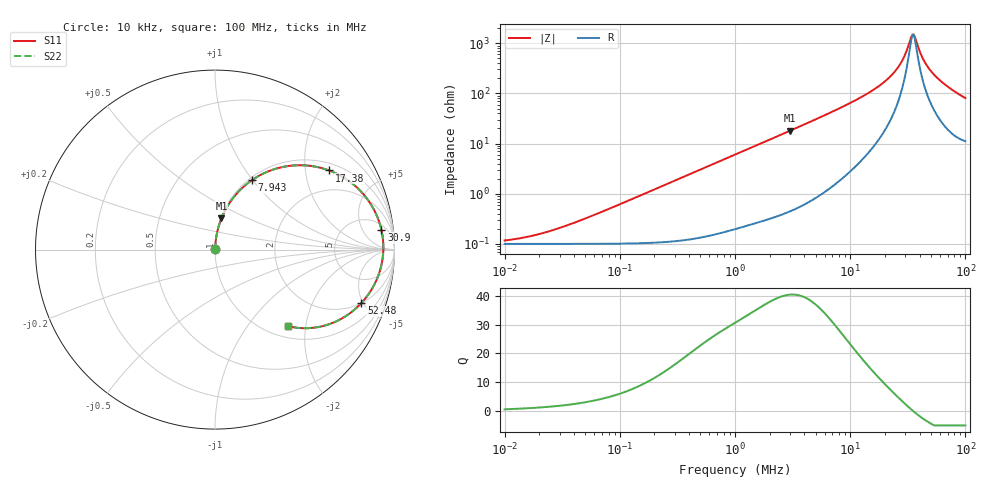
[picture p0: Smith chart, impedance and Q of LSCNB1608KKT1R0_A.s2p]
! LSCNB1608KKT1R0_A  S-PARAMETER MODEL  ( Standard Model )
! Model Generated by TAIYO YUDEN Corporation (http://www.ty-top.com)
! Version 1.0
! TAIYO YUDEN Control No. 170927
! Copyright(c) 2017 TAIYO YUDEN CO.,LTD. All Rights Reserved.
! Product Description (link to TY-COMPAS)
! https://ds.yuden.co.jp/TYCOMPAS/or/detail?pn=LSCNB1608KKT1R0MA&u=M
! Products Name : Inductors
! Characteristics :
!  Inductance : 1.0 [uH] , SRF(min) : - [Hz] , DC Resistance(max) : 123 [mOhm]
!  Rated Current : Saturation  2.0 [A] (dL = 30 [%]), Temp Rise  1.3 [A] (dT = 40 [degC])
!  Case Size : 1.6 x 0.8 / 0.063 x 0.031 [mm/inch] , Thickness : 1.0 / 0.039 [mm/inch]
!  (Conditions: Temperature = 25 [degC] , DC Bias Current = 0 [A])
! External Node Assignments :
!  1  o---GGG---o  2
! GND o---------o GND
! Frequency Range : 10kHz  -  100MHz  [ 402 STEP ]
# MHz S RI R 50
! Freq[MHz].  S11 Real  S11 Imag  S21 Real  S21 Imag  S12 Real  S12 Imag  S22 Real  S22 Imag
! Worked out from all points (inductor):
!   401 points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, 10 kHz to 100 MHz, reference 50 ohm
!   read as one part in series: L = 968 nH near 50.12 kHz
!   highest Q = 40.4 at 3.02 MHz (marker M1), where L = 954 nH
!   self-resonance near 35.2 MHz
!   S11 on the Smith chart (normalised r, x): 10 kHz: 1.00, +0.00; 7.943 MHz: 1.04, +0.99; 17.38 MHz: 1.23, +2.70; 30.9 MHz: 7, +13; 52.48 MHz: 2.01, -4.85; 100 MHz: 1.22, -1.59
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0.01  0.000999 0.000607  0.999 -0.000607  0.999 -0.000607  0.000999 0.000607
0.020417  0.001 0.00124  0.999 -0.00124  0.999 -0.00124  0.001 0.00124
0.046774  0.00101 0.00284  0.999 -0.00284  0.999 -0.00284  0.00101 0.00284
0.218776  0.00125 0.0133  0.9988 -0.0133  0.9988 -0.0133  0.00125 0.0133
1  0.00556 0.0598  0.9944 -0.0598  0.9944 -0.0598  0.00556 0.0598
3.019952  0.0358 0.1738  0.9642 -0.1738  0.9642 -0.1738  0.0358 0.1738
4.677351  0.0799 0.2582  0.9201 -0.2582  0.9201 -0.2582  0.0799 0.2582
7.943282  0.2058 0.387  0.7942 -0.387  0.7942 -0.387  0.2058 0.387
12.30269  0.4117 0.4662  0.5883 -0.4662  0.5883 -0.4662  0.4117 0.4662
17.37801  0.6357 0.4411  0.3643 -0.4411  0.3643 -0.4411  0.6357 0.4411
21.87762  0.7844 0.3518  0.2156 -0.3518  0.2156 -0.3518  0.7844 0.3518
26.91535  0.8874 0.2192  0.1126 -0.2192  0.1126 -0.2192  0.8874 0.2192
30.90295  0.9271 0.1101  0.0729 -0.1101  0.0729 -0.1101  0.9271 0.1101
33.88442  0.9375 0.0325  0.0625 -0.0325  0.0625 -0.0325  0.9375 0.0325
35.48134  0.9376 -0.00673  0.0624 0.00673  0.0624 0.00673  0.9376 -0.00673
37.15352  0.9343 -0.0457  0.0657 0.0457  0.0657 0.0457  0.9343 -0.0457
40.73803  0.9178 -0.1214  0.0822 0.1214  0.0822 0.1214  0.9178 -0.1214
43.65158  0.8973 -0.175  0.1027 0.175  0.1027 0.175  0.8973 -0.175
52.48075  0.8152 -0.2979  0.1848 0.2979  0.1848 0.2979  0.8152 -0.2979
60.25596  0.7342 -0.367  0.2658 0.367  0.2658 0.367  0.7342 -0.367
72.4436  0.6114 -0.4234  0.3886 0.4234  0.3886 0.4234  0.6114 -0.4234
100  0.4058 -0.4262  0.5942 0.4262  0.5942 0.4262  0.4058 -0.4262
